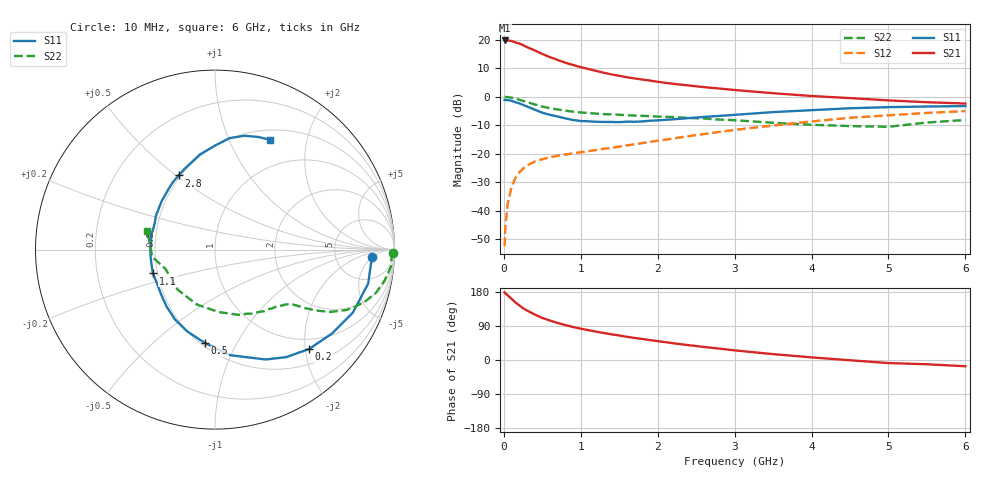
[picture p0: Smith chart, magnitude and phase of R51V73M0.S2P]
! SIEMENS Small Signal Semiconductors
! BFR183
! Si NPN RF Bipolar Junction Transistor in SOT23
! VCE = 1.75 V  IC = 3 mA
! Common Emitter S-Parameters:  May  1996
# GHz  S  MA  R  50
!  f  S11  S21  S12  S22
! GHz  MAG  ANG  MAG  ANG  MAG  ANG  MAG  ANG
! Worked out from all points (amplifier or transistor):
!   36 points, 10 MHz to 6 GHz, reference 50 ohm
!   highest |S21| = 19.7 dB at 10 MHz (marker M1)
!   |S21| within 3 dB of that: start of sweep to 359.1 MHz
!   unconditionally stable (mu >= 1): 1.225 GHz to 2.792 GHz
!   at 250 MHz: K = 0.30, MSG = 21.6 dB, |S12| = -25.2 dB
!   at 1.4 GHz: K = 1.06, MAG = 11.4 dB, |S12| = -17.9 dB
!   at 6 GHz: K = 0.91, MSG = 1.3 dB, |S12| = -5.0 dB
!   S11 on the Smith chart (normalised r, x): 10 MHz: 14, -5; 200 MHz: 0.78, -2.08; 500 MHz: 0.52, -0.75; 1.1 GHz: 0.47, -0.15; 2.8 GHz: 0.49, +0.51; 6 GHz: 0.62, +1.43
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0.01  0.8779 -2.6  9.664 178.4  0.0024 88.2  0.9937 -1.1
0.02  0.8727 -4.9  9.513 176.1  0.0053 88.9  0.9848 -2.1
0.05  0.8743 -12.5  9.663 170.6  0.0133 83.2  0.9857 -5.4
0.1  0.8448 -24.5  9.473 161.4  0.026 76.8  0.9596 -10.5
0.15  0.802 -35.7  8.923 152.1  0.0375 70.8  0.9289 -15.0
0.2  0.7625 -46.6  8.565 144.1  0.0469 66.5  0.8869 -18.9
0.25  0.7186 -56.5  7.993 136.9  0.055 61.8  0.8429 -22.2
0.3  0.6739 -65.3  7.389 130.6  0.0622 58.4  0.8052 -24.7
0.4  0.5936 -82.0  6.486 120.2  0.0727 53.3  0.7322 -28.3
0.5  0.5238 -96.1  5.601 110.9  0.08 50.2  0.6699 -30.6
0.6  0.4813 -108.8  4.927 104.0  0.0866 48.5  0.6276 -32.0
0.7  0.4483 -119.9  4.396 97.7  0.0922 47.5  0.5965 -33.1
0.8  0.4163 -130.5  3.936 92.2  0.0969 47.2  0.5686 -33.9
0.9  0.3905 -140.1  3.588 87.1  0.1019 47.6  0.5454 -34.6
1.1  0.3702 -159.0  3.05 78.7  0.1112 48.8  0.5162 -36.4
1.6  0.3648 167.0  2.189 61.2  0.1399 51.8  0.4739 -41.7
2.2  0.4013 137.8  1.68 44.3  0.1845 53.8  0.44 -51.2
2.8  0.4603 116.2  1.39 30.1  0.2415 51.8  0.3966 -64.4
3.5  0.5369 98.9  1.15 15.5  0.3125 45.9  0.3485 -86.7
4.5  0.6267 82.5  0.944 -0.7  0.4265 33.8  0.3052 -132.8
5.5  0.6726 68.9  0.799 -11.2  0.5194 20.4  0.3523 -173.5
6  0.6841 63.4  0.758 -16.5  0.5594 11.7  0.3903 164.5
